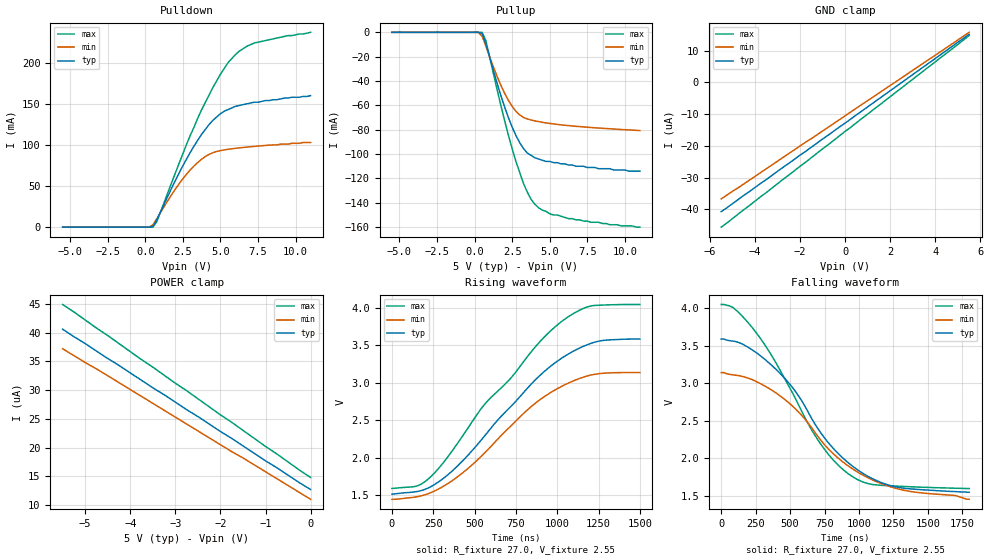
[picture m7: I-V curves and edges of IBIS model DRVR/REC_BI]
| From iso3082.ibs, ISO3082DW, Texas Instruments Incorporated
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|   Driver Output / Receiver Input Model
[Model]   DRVR/REC_BI
Model_type   I/O
| Signals   A,B
Vinl = 0.9V
Vinh = 2.8V
Vmeas = 1.7V   |Reference voltage for timing measurements
Cref = 50pF   |Timing specification test load capacitance value
Rref = 54   |Note: 54 Ohm load; single-ended configuration
|   Timing specification test load voltage
| variable   typ   min   max
C_comp   13.3pF   10.7pF   16.0pF
|   typ   min   max
[Temperature Range]   25.0   -40   85
[Voltage range]   5.0V   4.5V   5.5V
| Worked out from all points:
|   slope of the pulldown table from 0 to 0.75 V, typ, clamps not added: 89.2 ohm
|   slope of the pullup table from 0 to 0.75 V, typ, clamps not added: 79.1 ohm
|   rising waveform, R_fixture 27.0, V_fixture 2.55: 20-80 % time 518ns typ, 491ns min, 536ns max; typ from 1.51 V to 3.59 V
|   falling waveform, R_fixture 27.0, V_fixture 2.55: 20-80 % time 512ns typ, 567ns min, 464ns max; typ from 3.59 V to 1.54 V
[Pulldown]
|   Voltage   I(typ)   I(min)   I(max)
-5.5V     -28.1nA    -33.7nA    -24.1nA
250mV     123nA      21.1uA     -28.1nA
500mV     666uA      2.79mA     13.9uA
750mV     8.41mA     9.81mA     6.1mA
2.25V     65.9mA     52.8mA     77.8mA
3.25V     98.9mA     74.6mA     122mA
3.75V     113mA      82.7mA     143mA
4.5V      130mA      90.6mA     170mA
5.5V      143mA      94.7mA     200mA
6.25V     148mA      96.4mA     214mA
7.25V     152mA      98.2mA     224mA
11V       160mA      103mA      237mA
[Pullup]
|   Voltage   I(typ)   I(min)   I(max)
| Note that the[Pullup]voltage table is referenced to Vcc
| and is calculated using Vtable=Vcc - Vmeasured.
-5.5V     22.3nA     22.5nA     16.8nA
250mV     -132nA     -21.2uA    18.4nA
500mV     -700uA     -3.14mA    -13.9uA
750mV     -9.48mA    -11.3mA    -6.85mA
1.75V     -52mA      -43.5mA    -60.1mA
2.5V      -77.8mA    -60.8mA    -95.6mA
3.25V     -95.4mA    -69.9mA    -124mA
3.75V     -101mA     -72mA      -137mA
4V        -103mA     -72.7mA    -141mA
5V        -106mA     -74.8mA    -149mA
6.25V     -109mA     -76.6mA    -153mA
11V       -114mA     -80.7mA    -160mA
[GND_clamp]
|   Voltage  I(typ)   I(min)   I(max)
| Outputs in High Impedance (off)
-5.5V     -40.7uA    -36.7uA    -45.6uA
-1.75V    -21.7uA    -18.8uA    -25.1uA
-1.5V     -20.4uA    -17.7uA    -23.7uA
5.5V      15.2uA     15.8uA     14.8uA
[POWER_clamp]
|   Voltage  I(typ)   I(min)   I(max)
| Note that the [POWER_clamp] voltage table is referenced to Vcc
| and is calculated using Vtable = Vcc - Vmeasured.
| Outputs in Tri-state.
-5.5V     40.6uA     37.2uA     44.9uA
-4.75V    36.8uA     33.7uA     40.8uA
-1V       17.7uA     15.8uA     20.2uA
0V        12.7uA     11uA       14.8uA
[Ramp]
|   typ   min   max
dV/dt_r   0.91V/518ns   0.87V/492ns   0.95V/536ns
dV/dt_f   1.22V/524ns   0.99V/465ns   1.47V/569ns
R_load = 27ohm | Note: The measurement is on a single-ended configuration
|   with 54ohm line-to-line.
[Rising Waveform]
R_fixture = 27.0
V_fixture = 2.55
V_fixture_min = 2.276
V_fixture_max = 2.843
C_fixture = 0p
L_fixture = 0n
|   V(typ)   V(min)  V(max)
0s        1.514V     1.445V     1.59V
160ns     1.552V     1.483V     1.63V
240ns     1.62V      1.539V     1.758V
380ns     1.855V     1.718V     2.14V
560ns     2.29V      2.063V     2.712V
720ns     2.686V     2.426V     3.066V
840ns     2.978V     2.679V     3.408V
1.04us    3.349V     2.969V     3.842V
1.2us     3.525V     3.103V     4.026V
1.5us     3.586V     3.138V     4.047V
[Falling Waveform]
R_fixture = 27.0
V_fixture = 2.55
V_fixture_min = 2.276
V_fixture_max = 2.843
C_fixture = 0p
L_fixture = 0n
|   V(typ)   V(min)  V(max)
0s        3.586V     3.139V     4.047V
80ns      3.56V      3.111V     4.013V
160ns     3.513V     3.086V     3.877V
400ns     3.179V     2.865V     3.261V
560ns     2.833V     2.617V     2.715V
700ns     2.398V     2.293V     2.247V
920ns     1.941V     1.898V     1.794V
1.06us    1.762V     1.743V     1.663V
1.24us    1.628V     1.611V     1.629V
1.8us     1.544V     1.45V      1.594V
